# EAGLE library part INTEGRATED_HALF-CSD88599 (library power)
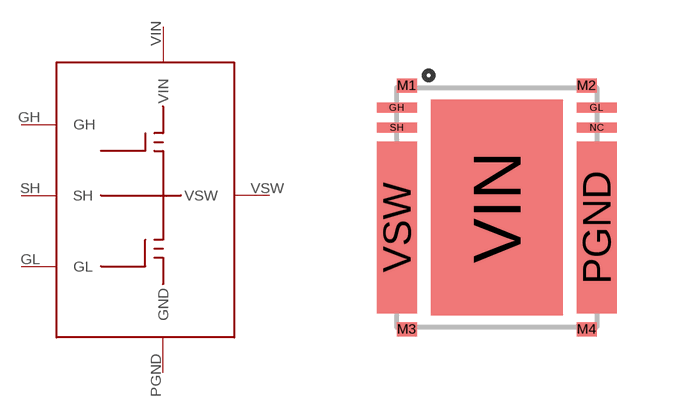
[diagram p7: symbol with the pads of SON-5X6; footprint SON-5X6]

Designator prefix -

## INTEGRATED_HALF-CSD88599SON  [SON-5X6]
GH  GH
GL  GL
PGND  GND
SH  SH
VIN  VIN
VSW  VSW

## Footprint SON-5X6 (pad centres in mm)
smd 1 x 0.25: GH -2.5,2.5; GL 2.5,2.5; NC 2.5,2; SH -2.5,2
smd 0.5 x 0.35: M1 -2.25,3.05; M2 2.25,3.05; M3 -2.25,-3.05; M4 2.25,-3.05
smd 1 x 4.3: PGND 2.5,-0.5; VSW -2.5,-0.5
smd 3.3 x 5.4: VIN 0,0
